(* states according to PackTags v3.0 *)
{attribute 'qualified_only'}
{attribute 'strict'}
TYPE E_PMLState :
(
	UNDEFINED		:=  0,
	CLEARING 		:=  1,
	STOPPED 		:=  2,
	STARTING 		:=  3,
	IDLE 			:=  4,
	SUSPENDED 		:=  5,
	EXECUTE 		:=  6,
	STOPPING	 	:=  7,
	ABORTING 		:=  8,
	ABORTED 		:=  9,
	HOLDING 		:= 10,
	HELD 			:= 11,
	UNHOLDING 		:= 12,
	SUSPENDING 		:= 13,
	UNSUSPENDING 	:= 14,
	RESETTING 		:= 15,
	COMPLETING 		:= 16,
	COMPLETE	 	:= 17
);
END_TYPE
